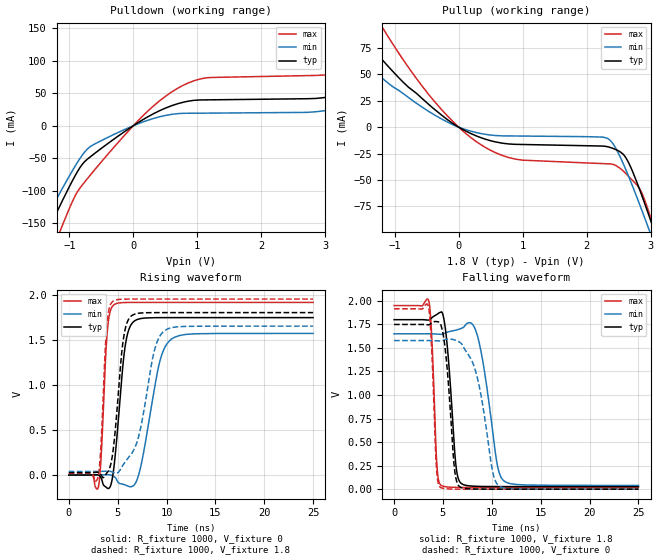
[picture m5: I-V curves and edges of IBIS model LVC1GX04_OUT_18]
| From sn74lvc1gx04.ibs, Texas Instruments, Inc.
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[Model]   LVC1GX04_OUT_18
Model_type  Output
Vref =   0
Rref =   1000
Cref =   30p
Vmeas =   0.9
| variable   typ   min   max
C_comp   9.95pF   6.40pF   16.08pF
| C_pullup   9.16pF   6.40pF   10.36pF
| C_pulldown   10.74pF   6.93pF   16.08pF
[Temperature Range]   40   100   -40
| Ambient temperature   25   85   -40
[Voltage range]   1.8   1.65   1.95
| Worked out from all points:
|   slope of the pulldown table from 0 to 0.27 V, typ, clamps not added: 16.8 ohm
|   slope of the pullup table from 0 to 0.27 V, typ, clamps not added: 33 ohm
|   rising waveform, R_fixture 1000, V_fixture 0: 20-80 % time 863ps typ, 1.55ns min, 502ps max; typ from 0 V to 1.74 V
|   falling waveform, R_fixture 1000, V_fixture 1.8: 20-80 % time 710ps typ, 1.27ns min, 425ps max; typ from 1.8 V to 0.027 V
|   rising waveform, R_fixture 1000, V_fixture 1.8: 20-80 % time 860ps typ, 1.68ns min, 500ps max; typ from 0.027 V to 1.8 V
|   falling waveform, R_fixture 1000, V_fixture 0: 20-80 % time 741ps typ, 1.56ns min, 428ps max; typ from 1.75 V to 0 V
[Pulldown]
| LVC1GX04_OUT_18
|   Voltage   I(typ)   I(min)   I(max)
-5.5V     -1.02A     -914.2mA   -1.211A
-1.49V    -194.3mA   -166.1mA   -248.7mA
-1.27V    -148.7mA   -125.7mA   -193.7mA
-1.11V    -116mA     -96.9mA    -154.1mA
-645mV    -45.9mA    -30.54mA   -72.92mA
690mV     33.84mA    18.58mA    57.6mA
3.205V    47.35mA    26.83mA    81.75mA
4.215V    79.09mA    21.52mA    130mA
4.445V    47.14mA    21.65mA    144.9mA
4.62V     44.43mA    21.75mA    152.8mA
5.01V     44.71mA    21.98mA    83.26mA
11V       50.71mA    25.31mA    93.17mA
[Pullup]
| LVC1GX04_OUT_18
|   Voltage   I(typ)   I(min)   I(max)
-5.5V     449.7mA    254mA      638.5mA
-2.225V   143.3mA    107.6mA    207.3mA
-1.755V   105.1mA    78.04mA    153.5mA
-1.195V   63.95mA    46.44mA    94.81mA
-375mV    16.75mA    11.48mA    24.15mA
420mV     -11.47mA   -6.842mA   -19.31mA
2.34V     -18.75mA   -11.19mA   -34.79mA
2.61V     -28.71mA   -39.94mA   -43.87mA
2.825V    -58.63mA   -72.76mA   -58mA
2.97V     -83.15mA   -96.31mA   -80.03mA
3.12V     -109.8mA   -121.4mA   -108.9mA
11V       -1.703A    -1.583A    -1.935A
[Ramp]
| LVC1GX04_OUT_18
| variable   typ   min   max
dV/dt_r   1.14/9.34E-10   1.02/1.66E-09   1.24/5.45E-10
dV/dt_f   1.11/7.58E-10   1.04/1.40E-09   1.20/4.49E-10
R_load = 1000
[Rising Waveform]
| LVC1GX04_OUT_18
R_fixture =   1000
C_fixture =   0
L_fixture =   0
V_fixture =   0
V_fixture_min = 0
V_fixture_max = 0
|   Time   V(typ)   V(min)   V(max)
0s        114pV      8.171nV    2.621nV
3.02ns    1.685mV    -212.7uV   -137.3mV
3.305ns   -30.1mV    678.1uV    189.2mV
3.945ns   -145.3mV   2.832mV    1.591V
4.635ns   100.4mV    -17.47mV   1.887V
5.735ns   1.4V       -108.5mV   1.912V
6.7ns     1.705V     -109.3mV   1.913V
9.28ns    1.744V     1.244V     1.913V
10.41ns   1.744V     1.498V     1.913V
24.99ns   1.744V     1.569V     1.913V
[Falling Waveform]
| LVC1GX04_OUT_18
R_fixture =   1000
C_fixture =   0
L_fixture =   0
V_fixture =   1.8
V_fixture_min = 1.65
V_fixture_max = 1.95
|   Time   V(typ)   V(min)   V(max)
0s        1.8V       1.65V      1.95V
3.555ns   1.796V     1.65V      1.998V
4.38ns    1.856V     1.647V     258.4mV
4.8ns     1.881V     1.644V     41.64mV
5.415ns   1.549V     1.666V     24.01mV
6.335ns   248.3mV    1.69V      19.24mV
6.835ns   63.93mV    1.706V     18.66mV
8.535ns   30.03mV    1.627V     18.24mV
11.21ns   27.48mV    89.22mV    18.21mV
24.99ns   27.29mV    39.58mV    18.21mV
[Rising Waveform]
| LVC1GX04_OUT_18
R_fixture =   1000
C_fixture =   0
L_fixture =   0
V_fixture =   1.8
V_fixture_min = 1.65
V_fixture_max = 1.95
|   Time   V(typ)   V(min)   V(max)
0s        27.26mV    39.51mV    18.19mV
2.97ns    30.07mV    39.35mV    -33.66mV
3.275ns   6.42mV     40.07mV    297.5mV
3.89ns    21.49mV    41.97mV    1.649V
4.525ns   262.2mV    30.85mV    1.925V
5.57ns    1.492V     113.3mV    1.949V
6.465ns   1.769V     241.9mV    1.95V
8.785ns   1.8V       1.389V     1.95V
9.835ns   1.8V       1.603V     1.95V
24.99ns   1.8V       1.65V      1.95V
[Falling Waveform]
| LVC1GX04_OUT_18
R_fixture =   1000
C_fixture =   0
L_fixture =   0
V_fixture =   0
V_fixture_min = 0
V_fixture_max = 0
|   Time   V(typ)   V(min)   V(max)
0s        1.749V     1.578V     1.916V
3.52ns    1.746V     1.578V     1.937V
4.325ns   1.78V      1.576V     246.7mV
4.72ns    1.761V     1.574V     20.71mV
5.335ns   1.389V     1.591V     4.592mV
6.195ns   205.5mV    1.585V     826.1uV
6.695ns   27.58mV    1.562V     347.9uV
8.4ns     1.411mV    1.232V     38.16uV
10.71ns   137.7uV    36.04mV    17.63uV
24.99ns   22.91uV    49.23uV    12.08uV
